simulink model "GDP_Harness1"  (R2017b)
settings: Solver=FixedStepDiscrete  StartTime=0.0  StopTime=2  FixedStep=0.01  RelTol=1e-3  EnableMultiTasking=on
undefined symbols (not defined in the file): sigbuilder_block

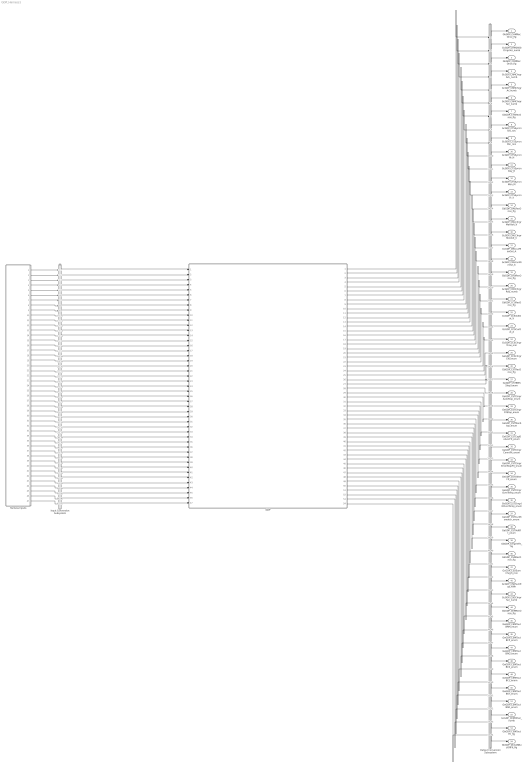
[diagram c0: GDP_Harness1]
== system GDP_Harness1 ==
  GDP : ModelReference  ModelNameDialog=GDP  SimulationMode=Normal  ModelReferenceVersion='M100C100'
  Harness Inputs : Subsystem  Tag=STV Subsys  LoadFcn=sigbuilder_block('load');  StartFcn=sigbuilder_block('start');  StopFcn=sigbuilder_block('stop');  ClipboardFcn=sigbuilder_block('clipboard');  mask(Sigbuilder block){tuvar=[0:10]}
      mask init:
      | if ~strcmp(get_param(bdroot(gcb),'SimulationStatus'),'stopped'),tuvar = sigbuilder_block('maskInit'); end
  Input Conversion Subsystem : Subsystem  Tag=__SLT_ICS__  Description=Signal spec. and routing
  Output Conversion Subsystem : Subsystem  Tag=__SLT_OCS__  Description=Signal spec. and routing
  GbGDP_CHMRecOnce_flg : Outport  OutDataTypeStr=boolean  PortDimensions=[1]
  GcGDP_CHM2600ChrgrVer_numb : Outport  Port=2  OutDataTypeStr=uint32  PortDimensions=[1]
  GbGDP_CRMRecOnce_flg : Outport  Port=3  OutDataTypeStr=boolean  PortDimensions=[1]
  GcGDP_CRMChrgrAck_numb : Outport  Port=4  OutDataTypeStr=uint8  PortDimensions=[1]
  GcGDP_CRMChrgrAr_numb : Outport  Port=5  OutDataTypeStr=uint32  PortDimensions=[1]
  GcGDP_CRMChrgrSer_numb : Outport  Port=6  OutDataTypeStr=uint32  PortDimensions=[1]
  GbGDP_CTSRecOnce_flg : Outport  Port=7  OutDataTypeStr=boolean  PortDimensions=[1]
  GcGDP_CTSSyncnSec_sec : Outport  Port=8  OutDataTypeStr=uint8  PortDimensions=[1]
  GcGDP_CTSSyncnMin_min : Outport  Port=9  OutDataTypeStr=uint8  PortDimensions=[1]
  GcGDP_CTSSyncnHr_H : Outport  Port=10  OutDataTypeStr=uint8  PortDimensions=[1]
  GcGDP_CTSSyncnDay_D : Outport  Port=11  OutDataTypeStr=uint8  PortDimensions=[1]
  GcGDP_CTSSyncnMon_M : Outport  Port=12  OutDataTypeStr=uint8  PortDimensions=[1]
  GcGDP_CTSSyncnYr_Y : Outport  Port=13  OutDataTypeStr=uint16  PortDimensions=[1]
  GbGDP_CMLRecOnce_flg : Outport  Port=14  OutDataTypeStr=boolean  PortDimensions=[1]
  GcGDP_CMLChrgrMaxVolt_V : Outport  Port=15  OutDataTypeStr=single  PortDimensions=[1]
  GcGDP_CMLChrgrMinVolt_V : Outport  Port=16  OutDataTypeStr=single  PortDimensions=[1]
  GcGDP_CMLCurMaxOut_A : Outport  Port=17  OutDataTypeStr=single  PortDimensions=[1]
  GcGDP_CMLCurMinOut_A : Outport  Port=18  OutDataTypeStr=single  PortDimensions=[1]
  GbGDP_CRORecOnce_flg : Outport  Port=19  OutDataTypeStr=boolean  PortDimensions=[1]
  GcGDP_CROChrgrRdy_numb : Outport  Port=20  OutDataTypeStr=uint8  PortDimensions=[1]
  GbGDP_CCSRecOnce_flg : Outport  Port=21  OutDataTypeStr=boolean  PortDimensions=[1]
  GcGDP_CCSVoltOut_V : Outport  Port=22  OutDataTypeStr=single  PortDimensions=[1]
  GcGDP_CCSCurOut_A : Outport  Port=23  OutDataTypeStr=single  PortDimensions=[1]
  GcGDP_CCSChrgrTime_min : Outport  Port=24  OutDataTypeStr=single  PortDimensions=[1]
  GeGDP_CCSChrgrEN_enum : Outport  Port=25  OutDataTypeStr=uint8  PortDimensions=[1]
  GbGDP_CSTRecOnce_flg : Outport  Port=26  OutDataTypeStr=boolean  PortDimensions=[1]
  GeGDP_CSTBMSStop_enum : Outport  Port=27  OutDataTypeStr=uint8  PortDimensions=[1]
  GeGDP_CSTChrgrAutoStop_enum : Outport  Port=28  OutDataTypeStr=uint8  PortDimensions=[1]
  GeGDP_CSTChrgrFltStop_enum : Outport  Port=29  OutDataTypeStr=uint8  PortDimensions=[1]
  GeGDP_CSTManStop_enum : Outport  Port=30  OutDataTypeStr=uint8  PortDimensions=[1]
  GeGDP_CSTCapDeliverFlt_enum : Outport  Port=31  OutDataTypeStr=uint8  PortDimensions=[1]
  GeGDP_CSTChrgrConntFlt_enum : Outport  Port=32  OutDataTypeStr=uint8  PortDimensions=[1]
  GeGDP_CSTChrgrEmerStopFlt_enum : Outport  Port=33  OutDataTypeStr=uint8  PortDimensions=[1]
  GeGDP_CSTOtherFlt_enum : Outport  Port=34  OutDataTypeStr=uint8  PortDimensions=[1]
  GeGDP_CSTChrgrOverTemp_enum : Outport  Port=35  OutDataTypeStr=uint8  PortDimensions=[1]
  GeGDP_CSTChrgrIntOverTemp_enum : Outport  Port=36  OutDataTypeStr=uint8  PortDimensions=[1]
  GeGDP_CSTCurMismatch_enum : Outport  Port=37  OutDataTypeStr=uint8  PortDimensions=[1]
  GeGDP_CSTVoltFlt_enum : Outport  Port=38  OutDataTypeStr=uint8  PortDimensions=[1]
  GbGDP_ChrgrInFlt_flg : Outport  Port=39  OutDataTypeStr=boolean  PortDimensions=[1]
  GbGDP_CSDRecOnce_flg : Outport  Port=40  OutDataTypeStr=boolean  PortDimensions=[1]
  GcGDP_CSDSumChrgTi_min : Outport  Port=41  OutDataTypeStr=single  PortDimensions=[1]
  GcGDP_CSDSumEgy_kWh : Outport  Port=42  OutDataTypeStr=single  PortDimensions=[1]
  GcGDP_CSDChrgrSer_numb : Outport  Port=43  OutDataTypeStr=uint32  PortDimensions=[1]
  GbGDP_CEMRecOnce_flg : Outport  Port=44  OutDataTypeStr=boolean  PortDimensions=[1]
  GeGDP_CEMToutBRM_enum : Outport  Port=45  OutDataTypeStr=uint8  PortDimensions=[1]
  GeGDP_CEMToutBCP_enum : Outport  Port=46  OutDataTypeStr=uint8  PortDimensions=[1]
  GeGDP_CEMToutBRO_enum : Outport  Port=47  OutDataTypeStr=uint8  PortDimensions=[1]
  GeGDP_CEMToutBCS_enum : Outport  Port=48  OutDataTypeStr=uint8  PortDimensions=[1]
  GeGDP_CEMToutBCL_enum : Outport  Port=49  OutDataTypeStr=uint8  PortDimensions=[1]
  GeGDP_CEMToutBST_enum : Outport  Port=50  OutDataTypeStr=uint8  PortDimensions=[1]
  GeGDP_CEMToutBSD_enum : Outport  Port=51  OutDataTypeStr=uint8  PortDimensions=[1]
  GcGDP_CEMOther_numb : Outport  Port=52  OutDataTypeStr=uint8  PortDimensions=[1]
  GbGDP_CEMToutFlt_flg : Outport  Port=53  OutDataTypeStr=boolean  PortDimensions=[1]
  GbGDP_DCCANBusOffFlt_flg : Outport  Port=54  OutDataTypeStr=boolean  PortDimensions=[1]
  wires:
  Harness Inputs/1(GcISP_2600ChrgrVer_numb) -> Input Conversion Subsystem/1(Inport_1)
  Harness Inputs/2(GcISP_2560ChrgrAck_numb) -> Input Conversion Subsystem/2(Inport_2)
  Harness Inputs/3(GcISP_2561ChrgrSer_numb) -> Input Conversion Subsystem/3(Inport_3)
  Harness Inputs/4(GcISP_2562ChrgrAr_numb) -> Input Conversion Subsystem/4(Inport_4)
  Harness Inputs/5(GcISP_2823SyncnSec_sec) -> Input Conversion Subsystem/5(Inport_5)
  Harness Inputs/6(GcISP_2823SyncnMin_min) -> Input Conversion Subsystem/6(Inport_6)
  Harness Inputs/7(GcISP_2823SyncnHr_H) -> Input Conversion Subsystem/7(Inport_7)
  Harness Inputs/8(GcISP_2823SyncnDay_D) -> Input Conversion Subsystem/8(Inport_8)
  Harness Inputs/9(GcISP_2823SyncnMon_M) -> Input Conversion Subsystem/9(Inport_9)
  Harness Inputs/10(GcISP_2823SyncnYr_Y) -> Input Conversion Subsystem/10(Inport_10)
  Harness Inputs/11(GcISP_2824ChrgrMaxVolt_V) -> Input Conversion Subsystem/11(Inport_11)
  Harness Inputs/12(GcISP_2825ChrgrMinVolt_V) -> Input Conversion Subsystem/12(Inport_12)
  Harness Inputs/13(GcISP_2826ChrgrMaxCur_A) -> Input Conversion Subsystem/13(Inport_13)
  Harness Inputs/14(GcISP_2827ChrgrMinCur_A) -> Input Conversion Subsystem/14(Inport_14)
  Harness Inputs/15(GcISP_2830ChrgrRdy_numb) -> Input Conversion Subsystem/15(Inport_15)
  Harness Inputs/16(GcISP_3081ChrgrVolt_V) -> Input Conversion Subsystem/16(Inport_16)
  Harness Inputs/17(GcISP_3082ChrgrCur_A) -> Input Conversion Subsystem/17(Inport_17)
  Harness Inputs/18(GcISP_3083ChrgTi_min) -> Input Conversion Subsystem/18(Inport_18)
  Harness Inputs/19(GeISP_3929ChrgrRdy_enum) -> Input Conversion Subsystem/19(Inport_19)
  Harness Inputs/20(GeISP_3521BMSStop_enum) -> Input Conversion Subsystem/20(Inport_20)
  Harness Inputs/21(GeISP_3521ChrgrAuto_enum) -> Input Conversion Subsystem/21(Inport_21)
  Harness Inputs/22(GeISP_3521ChrgrFlt_enum) -> Input Conversion Subsystem/22(Inport_22)
  Harness Inputs/23(GeISP_3521ManStop_enum) -> Input Conversion Subsystem/23(Inport_23)
  Harness Inputs/24(GeISP_3522CapDeliverFlt_enum) -> Input Conversion Subsystem/24(Inport_24)
  Harness Inputs/25(GeISP_3522ChrgrConntFlt_enum) -> Input Conversion Subsystem/25(Inport_25)
  Harness Inputs/26(GeISP_3522ChrgrEmerStopFlt_enum) -> Input Conversion Subsystem/26(Inport_26)
  Harness Inputs/27(GeISP_3522OtherFlt_enum) -> Input Conversion Subsystem/27(Inport_27)
  Harness Inputs/28(GeISP_3522ChrgrOverTemp_enum) -> Input Conversion Subsystem/28(Inport_28)
  Harness Inputs/29(GeISP_3522ChrgrIntOverTemp_enum) -> Input Conversion Subsystem/29(Inport_29)
  Harness Inputs/30(GeISP_3523CurMismatch_enum) -> Input Conversion Subsystem/30(Inport_30)
  Harness Inputs/31(GeISP_3523VoltFlt_enum) -> Input Conversion Subsystem/31(Inport_31)
  Harness Inputs/32(GcISP_3611SumChrgTi_min) -> Input Conversion Subsystem/32(Inport_32)
  Harness Inputs/33(GcISP_3612SumEgy_kWh) -> Input Conversion Subsystem/33(Inport_33)
  Harness Inputs/34(GcISP_3613ChrgrSer_numb) -> Input Conversion Subsystem/34(Inport_34)
  Harness Inputs/35(GeISP_3921ToutBRM_enum) -> Input Conversion Subsystem/35(Inport_35)
  Harness Inputs/36(GeISP_3922ToutBCP_enum) -> Input Conversion Subsystem/36(Inport_36)
  Harness Inputs/37(GeISP_3923ToutBRO_enum) -> Input Conversion Subsystem/37(Inport_37)
  Harness Inputs/38(GeISP_3924ToutBCS_enum) -> Input Conversion Subsystem/38(Inport_38)
  Harness Inputs/39(GeISP_3925ToutBCL_enum) -> Input Conversion Subsystem/39(Inport_39)
  Harness Inputs/40(GeISP_3926ToutBST_enum) -> Input Conversion Subsystem/40(Inport_40)
  Harness Inputs/41(GeISP_3927ToutBSD_enum) -> Input Conversion Subsystem/41(Inport_41)
  Harness Inputs/42(GcISP_CEMOther_numb) -> Input Conversion Subsystem/42(Inport_42)
  Harness Inputs/43(GeDCC_DCConnSt_enum) -> Input Conversion Subsystem/43(Inport_43)
  Harness Inputs/44(GbISP_DCCANBusOffFlt_flg) -> Input Conversion Subsystem/44(Inport_44)
  Harness Inputs/45(GbISP_DCChrgCanNetStatus_flg) -> Input Conversion Subsystem/45(Inport_45)
  Harness Inputs/46(GeLDP_CC2St_enum) -> Input Conversion Subsystem/46(Inport_46)
  Harness Inputs/47(GbLDP_DC12VSply_flg) -> Input Conversion Subsystem/47(Inport_47)
  Output Conversion Subsystem/1(Outport_1) -> GbGDP_CHMRecOnce_flg/1
  Output Conversion Subsystem/2(Outport_2) -> GcGDP_CHM2600ChrgrVer_numb/1
  Output Conversion Subsystem/3(Outport_3) -> GbGDP_CRMRecOnce_flg/1
  Output Conversion Subsystem/4(Outport_4) -> GcGDP_CRMChrgrAck_numb/1
  Output Conversion Subsystem/5(Outport_5) -> GcGDP_CRMChrgrAr_numb/1
  Output Conversion Subsystem/6(Outport_6) -> GcGDP_CRMChrgrSer_numb/1
  Output Conversion Subsystem/7(Outport_7) -> GbGDP_CTSRecOnce_flg/1
  Output Conversion Subsystem/8(Outport_8) -> GcGDP_CTSSyncnSec_sec/1
  Output Conversion Subsystem/9(Outport_9) -> GcGDP_CTSSyncnMin_min/1
  Output Conversion Subsystem/10(Outport_10) -> GcGDP_CTSSyncnHr_H/1
  Output Conversion Subsystem/11(Outport_11) -> GcGDP_CTSSyncnDay_D/1
  Output Conversion Subsystem/12(Outport_12) -> GcGDP_CTSSyncnMon_M/1
  Output Conversion Subsystem/13(Outport_13) -> GcGDP_CTSSyncnYr_Y/1
  Output Conversion Subsystem/14(Outport_14) -> GbGDP_CMLRecOnce_flg/1
  Output Conversion Subsystem/15(Outport_15) -> GcGDP_CMLChrgrMaxVolt_V/1
  Output Conversion Subsystem/16(Outport_16) -> GcGDP_CMLChrgrMinVolt_V/1
  Output Conversion Subsystem/17(Outport_17) -> GcGDP_CMLCurMaxOut_A/1
  Output Conversion Subsystem/18(Outport_18) -> GcGDP_CMLCurMinOut_A/1
  Output Conversion Subsystem/19(Outport_19) -> GbGDP_CRORecOnce_flg/1
  Output Conversion Subsystem/20(Outport_20) -> GcGDP_CROChrgrRdy_numb/1
  Output Conversion Subsystem/21(Outport_21) -> GbGDP_CCSRecOnce_flg/1
  Output Conversion Subsystem/22(Outport_22) -> GcGDP_CCSVoltOut_V/1
  Output Conversion Subsystem/23(Outport_23) -> GcGDP_CCSCurOut_A/1
  Output Conversion Subsystem/24(Outport_24) -> GcGDP_CCSChrgrTime_min/1
  Output Conversion Subsystem/25(Outport_25) -> GeGDP_CCSChrgrEN_enum/1
  Output Conversion Subsystem/26(Outport_26) -> GbGDP_CSTRecOnce_flg/1
  Output Conversion Subsystem/27(Outport_27) -> GeGDP_CSTBMSStop_enum/1
  Output Conversion Subsystem/28(Outport_28) -> GeGDP_CSTChrgrAutoStop_enum/1
  Output Conversion Subsystem/29(Outport_29) -> GeGDP_CSTChrgrFltStop_enum/1
  Output Conversion Subsystem/30(Outport_30) -> GeGDP_CSTManStop_enum/1
  Output Conversion Subsystem/31(Outport_31) -> GeGDP_CSTCapDeliverFlt_enum/1
  Output Conversion Subsystem/32(Outport_32) -> GeGDP_CSTChrgrConntFlt_enum/1
  Output Conversion Subsystem/33(Outport_33) -> GeGDP_CSTChrgrEmerStopFlt_enum/1
  Output Conversion Subsystem/34(Outport_34) -> GeGDP_CSTOtherFlt_enum/1
  Output Conversion Subsystem/35(Outport_35) -> GeGDP_CSTChrgrOverTemp_enum/1
  Output Conversion Subsystem/36(Outport_36) -> GeGDP_CSTChrgrIntOverTemp_enum/1
  Output Conversion Subsystem/37(Outport_37) -> GeGDP_CSTCurMismatch_enum/1
  Output Conversion Subsystem/38(Outport_38) -> GeGDP_CSTVoltFlt_enum/1
  Output Conversion Subsystem/39(Outport_39) -> GbGDP_ChrgrInFlt_flg/1
  Output Conversion Subsystem/40(Outport_40) -> GbGDP_CSDRecOnce_flg/1
  Output Conversion Subsystem/41(Outport_41) -> GcGDP_CSDSumChrgTi_min/1
  Output Conversion Subsystem/42(Outport_42) -> GcGDP_CSDSumEgy_kWh/1
  Output Conversion Subsystem/43(Outport_43) -> GcGDP_CSDChrgrSer_numb/1
  Output Conversion Subsystem/44(Outport_44) -> GbGDP_CEMRecOnce_flg/1
  Output Conversion Subsystem/45(Outport_45) -> GeGDP_CEMToutBRM_enum/1
  Output Conversion Subsystem/46(Outport_46) -> GeGDP_CEMToutBCP_enum/1
  Output Conversion Subsystem/47(Outport_47) -> GeGDP_CEMToutBRO_enum/1
  Output Conversion Subsystem/48(Outport_48) -> GeGDP_CEMToutBCS_enum/1
  Output Conversion Subsystem/49(Outport_49) -> GeGDP_CEMToutBCL_enum/1
  Output Conversion Subsystem/50(Outport_50) -> GeGDP_CEMToutBST_enum/1
  Output Conversion Subsystem/51(Outport_51) -> GeGDP_CEMToutBSD_enum/1
  Output Conversion Subsystem/52(Outport_52) -> GcGDP_CEMOther_numb/1
  Output Conversion Subsystem/53(Outport_53) -> GbGDP_CEMToutFlt_flg/1
  Output Conversion Subsystem/54(Outport_54) -> GbGDP_DCCANBusOffFlt_flg/1
  Input Conversion Subsystem/1(Outport_1) -> GDP/1
  Input Conversion Subsystem/2(Outport_2) -> GDP/2
  Input Conversion Subsystem/3(Outport_3) -> GDP/3
  Input Conversion Subsystem/4(Outport_4) -> GDP/4
  Input Conversion Subsystem/5(Outport_5) -> GDP/5
  Input Conversion Subsystem/6(Outport_6) -> GDP/6
  Input Conversion Subsystem/7(Outport_7) -> GDP/7
  Input Conversion Subsystem/8(Outport_8) -> GDP/8
  Input Conversion Subsystem/9(Outport_9) -> GDP/9
  Input Conversion Subsystem/10(Outport_10) -> GDP/10
  Input Conversion Subsystem/11(Outport_11) -> GDP/11
  Input Conversion Subsystem/12(Outport_12) -> GDP/12
  Input Conversion Subsystem/13(Outport_13) -> GDP/13
  Input Conversion Subsystem/14(Outport_14) -> GDP/14
  Input Conversion Subsystem/15(Outport_15) -> GDP/15
  Input Conversion Subsystem/16(Outport_16) -> GDP/16
  Input Conversion Subsystem/17(Outport_17) -> GDP/17
  Input Conversion Subsystem/18(Outport_18) -> GDP/18
  Input Conversion Subsystem/19(Outport_19) -> GDP/19
  Input Conversion Subsystem/20(Outport_20) -> GDP/20
  Input Conversion Subsystem/21(Outport_21) -> GDP/21
  Input Conversion Subsystem/22(Outport_22) -> GDP/22
  Input Conversion Subsystem/23(Outport_23) -> GDP/23
  Input Conversion Subsystem/24(Outport_24) -> GDP/24
  Input Conversion Subsystem/25(Outport_25) -> GDP/25
  Input Conversion Subsystem/26(Outport_26) -> GDP/26
  Input Conversion Subsystem/27(Outport_27) -> GDP/27
  Input Conversion Subsystem/28(Outport_28) -> GDP/28
  Input Conversion Subsystem/29(Outport_29) -> GDP/29
  Input Conversion Subsystem/30(Outport_30) -> GDP/30
  Input Conversion Subsystem/31(Outport_31) -> GDP/31
  Input Conversion Subsystem/32(Outport_32) -> GDP/32
  Input Conversion Subsystem/33(Outport_33) -> GDP/33
  Input Conversion Subsystem/34(Outport_34) -> GDP/34
  Input Conversion Subsystem/35(Outport_35) -> GDP/35
  Input Conversion Subsystem/36(Outport_36) -> GDP/36
  Input Conversion Subsystem/37(Outport_37) -> GDP/37
  Input Conversion Subsystem/38(Outport_38) -> GDP/38
  Input Conversion Subsystem/39(Outport_39) -> GDP/39
  Input Conversion Subsystem/40(Outport_40) -> GDP/40
  Input Conversion Subsystem/41(Outport_41) -> GDP/41
  Input Conversion Subsystem/42(Outport_42) -> GDP/42
  Input Conversion Subsystem/43(Outport_43) -> GDP/43
  Input Conversion Subsystem/44(Outport_44) -> GDP/44
  Input Conversion Subsystem/45(Outport_45) -> GDP/45
  Input Conversion Subsystem/46(Outport_46) -> GDP/46
  Input Conversion Subsystem/47(Outport_47) -> GDP/47
  GDP/1 -> Output Conversion Subsystem/1(Inport_1)
  GDP/2 -> Output Conversion Subsystem/2(Inport_2)
  GDP/3 -> Output Conversion Subsystem/3(Inport_3)
  GDP/4 -> Output Conversion Subsystem/4(Inport_4)
  GDP/5 -> Output Conversion Subsystem/5(Inport_5)
  GDP/6 -> Output Conversion Subsystem/6(Inport_6)
  GDP/7 -> Output Conversion Subsystem/7(Inport_7)
  GDP/8 -> Output Conversion Subsystem/8(Inport_8)
  GDP/9 -> Output Conversion Subsystem/9(Inport_9)
  GDP/10 -> Output Conversion Subsystem/10(Inport_10)
  GDP/11 -> Output Conversion Subsystem/11(Inport_11)
  GDP/12 -> Output Conversion Subsystem/12(Inport_12)
  GDP/13 -> Output Conversion Subsystem/13(Inport_13)
  GDP/14 -> Output Conversion Subsystem/14(Inport_14)
  GDP/15 -> Output Conversion Subsystem/15(Inport_15)
  GDP/16 -> Output Conversion Subsystem/16(Inport_16)
  GDP/17 -> Output Conversion Subsystem/17(Inport_17)
  GDP/18 -> Output Conversion Subsystem/18(Inport_18)
  GDP/19 -> Output Conversion Subsystem/19(Inport_19)
  GDP/20 -> Output Conversion Subsystem/20(Inport_20)
  GDP/21 -> Output Conversion Subsystem/21(Inport_21)
  GDP/22 -> Output Conversion Subsystem/22(Inport_22)
  GDP/23 -> Output Conversion Subsystem/23(Inport_23)
  GDP/24 -> Output Conversion Subsystem/24(Inport_24)
  GDP/25 -> Output Conversion Subsystem/25(Inport_25)
  GDP/26 -> Output Conversion Subsystem/26(Inport_26)
  GDP/27 -> Output Conversion Subsystem/27(Inport_27)
  GDP/28 -> Output Conversion Subsystem/28(Inport_28)
  GDP/29 -> Output Conversion Subsystem/29(Inport_29)
  GDP/30 -> Output Conversion Subsystem/30(Inport_30)
  GDP/31 -> Output Conversion Subsystem/31(Inport_31)
  GDP/32 -> Output Conversion Subsystem/32(Inport_32)
  GDP/33 -> Output Conversion Subsystem/33(Inport_33)
  GDP/34 -> Output Conversion Subsystem/34(Inport_34)
  GDP/35 -> Output Conversion Subsystem/35(Inport_35)
  GDP/36 -> Output Conversion Subsystem/36(Inport_36)
  GDP/37 -> Output Conversion Subsystem/37(Inport_37)
  GDP/38 -> Output Conversion Subsystem/38(Inport_38)
  GDP/39 -> Output Conversion Subsystem/39(Inport_39)
  GDP/40 -> Output Conversion Subsystem/40(Inport_40)
  GDP/41 -> Output Conversion Subsystem/41(Inport_41)
  GDP/42 -> Output Conversion Subsystem/42(Inport_42)
  GDP/43 -> Output Conversion Subsystem/43(Inport_43)
  GDP/44 -> Output Conversion Subsystem/44(Inport_44)
  GDP/45 -> Output Conversion Subsystem/45(Inport_45)
  GDP/46 -> Output Conversion Subsystem/46(Inport_46)
  GDP/47 -> Output Conversion Subsystem/47(Inport_47)
  GDP/48 -> Output Conversion Subsystem/48(Inport_48)
  GDP/49 -> Output Conversion Subsystem/49(Inport_49)
  GDP/50 -> Output Conversion Subsystem/50(Inport_50)
  GDP/51 -> Output Conversion Subsystem/51(Inport_51)
  GDP/52 -> Output Conversion Subsystem/52(Inport_52)
  GDP/53 -> Output Conversion Subsystem/53(Inport_53)
  GDP/54 -> Output Conversion Subsystem/54(Inport_54)

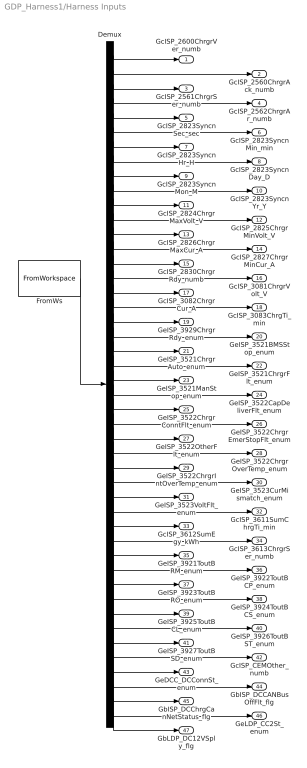
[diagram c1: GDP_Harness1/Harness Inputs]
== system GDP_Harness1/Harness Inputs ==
  Demux : Demux  Tag=STV Demux  Outputs=47
  FromWs : FromWorkspace  Tag=STV FromWs  VariableName=tuvar  SampleTime=0
  GcISP_2600ChrgrVer_numb : Outport  Tag=STV Outport
  GcISP_2560ChrgrAck_numb : Outport  Tag=STV Outport  Port=2
  GcISP_2561ChrgrSer_numb : Outport  Tag=STV Outport  Port=3
  GcISP_2562ChrgrAr_numb : Outport  Tag=STV Outport  Port=4
  GcISP_2823SyncnSec_sec : Outport  Tag=STV Outport  Port=5
  GcISP_2823SyncnMin_min : Outport  Tag=STV Outport  Port=6
  GcISP_2823SyncnHr_H : Outport  Tag=STV Outport  Port=7
  GcISP_2823SyncnDay_D : Outport  Tag=STV Outport  Port=8
  GcISP_2823SyncnMon_M : Outport  Tag=STV Outport  Port=9
  GcISP_2823SyncnYr_Y : Outport  Tag=STV Outport  Port=10
  GcISP_2824ChrgrMaxVolt_V : Outport  Tag=STV Outport  Port=11
  GcISP_2825ChrgrMinVolt_V : Outport  Tag=STV Outport  Port=12
  GcISP_2826ChrgrMaxCur_A : Outport  Tag=STV Outport  Port=13
  GcISP_2827ChrgrMinCur_A : Outport  Tag=STV Outport  Port=14
  GcISP_2830ChrgrRdy_numb : Outport  Tag=STV Outport  Port=15
  GcISP_3081ChrgrVolt_V : Outport  Tag=STV Outport  Port=16
  GcISP_3082ChrgrCur_A : Outport  Tag=STV Outport  Port=17
  GcISP_3083ChrgTi_min : Outport  Tag=STV Outport  Port=18
  GeISP_3929ChrgrRdy_enum : Outport  Tag=STV Outport  Port=19
  GeISP_3521BMSStop_enum : Outport  Tag=STV Outport  Port=20
  GeISP_3521ChrgrAuto_enum : Outport  Tag=STV Outport  Port=21
  GeISP_3521ChrgrFlt_enum : Outport  Tag=STV Outport  Port=22
  GeISP_3521ManStop_enum : Outport  Tag=STV Outport  Port=23
  GeISP_3522CapDeliverFlt_enum : Outport  Tag=STV Outport  Port=24
  GeISP_3522ChrgrConntFlt_enum : Outport  Tag=STV Outport  Port=25
  GeISP_3522ChrgrEmerStopFlt_enum : Outport  Tag=STV Outport  Port=26
  GeISP_3522OtherFlt_enum : Outport  Tag=STV Outport  Port=27
  GeISP_3522ChrgrOverTemp_enum : Outport  Tag=STV Outport  Port=28
  GeISP_3522ChrgrIntOverTemp_enum : Outport  Tag=STV Outport  Port=29
  GeISP_3523CurMismatch_enum : Outport  Tag=STV Outport  Port=30
  GeISP_3523VoltFlt_enum : Outport  Tag=STV Outport  Port=31
  GcISP_3611SumChrgTi_min : Outport  Tag=STV Outport  Port=32
  GcISP_3612SumEgy_kWh : Outport  Tag=STV Outport  Port=33
  GcISP_3613ChrgrSer_numb : Outport  Tag=STV Outport  Port=34
  GeISP_3921ToutBRM_enum : Outport  Tag=STV Outport  Port=35
  GeISP_3922ToutBCP_enum : Outport  Tag=STV Outport  Port=36
  GeISP_3923ToutBRO_enum : Outport  Tag=STV Outport  Port=37
  GeISP_3924ToutBCS_enum : Outport  Tag=STV Outport  Port=38
  GeISP_3925ToutBCL_enum : Outport  Tag=STV Outport  Port=39
  GeISP_3926ToutBST_enum : Outport  Tag=STV Outport  Port=40
  GeISP_3927ToutBSD_enum : Outport  Tag=STV Outport  Port=41
  GcISP_CEMOther_numb : Outport  Tag=STV Outport  Port=42
  GeDCC_DCConnSt_enum : Outport  Tag=STV Outport  Port=43
  GbISP_DCCANBusOffFlt_flg : Outport  Tag=STV Outport  Port=44
  GbISP_DCChrgCanNetStatus_flg : Outport  Tag=STV Outport  Port=45
  GeLDP_CC2St_enum : Outport  Tag=STV Outport  Port=46
  GbLDP_DC12VSply_flg : Outport  Tag=STV Outport  Port=47
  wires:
  FromWs/1 -> Demux/1
  Demux/1 -> GcISP_2600ChrgrVer_numb/1
  Demux/2 -> GcISP_2560ChrgrAck_numb/1
  Demux/3 -> GcISP_2561ChrgrSer_numb/1
  Demux/4 -> GcISP_2562ChrgrAr_numb/1
  Demux/5 -> GcISP_2823SyncnSec_sec/1
  Demux/6 -> GcISP_2823SyncnMin_min/1
  Demux/7 -> GcISP_2823SyncnHr_H/1
  Demux/8 -> GcISP_2823SyncnDay_D/1
  Demux/9 -> GcISP_2823SyncnMon_M/1
  Demux/10 -> GcISP_2823SyncnYr_Y/1
  Demux/11 -> GcISP_2824ChrgrMaxVolt_V/1
  Demux/12 -> GcISP_2825ChrgrMinVolt_V/1
  Demux/13 -> GcISP_2826ChrgrMaxCur_A/1
  Demux/14 -> GcISP_2827ChrgrMinCur_A/1
  Demux/15 -> GcISP_2830ChrgrRdy_numb/1
  Demux/16 -> GcISP_3081ChrgrVolt_V/1
  Demux/17 -> GcISP_3082ChrgrCur_A/1
  Demux/18 -> GcISP_3083ChrgTi_min/1
  Demux/19 -> GeISP_3929ChrgrRdy_enum/1
  Demux/20 -> GeISP_3521BMSStop_enum/1
  Demux/21 -> GeISP_3521ChrgrAuto_enum/1
  Demux/22 -> GeISP_3521ChrgrFlt_enum/1
  Demux/23 -> GeISP_3521ManStop_enum/1
  Demux/24 -> GeISP_3522CapDeliverFlt_enum/1
  Demux/25 -> GeISP_3522ChrgrConntFlt_enum/1
  Demux/26 -> GeISP_3522ChrgrEmerStopFlt_enum/1
  Demux/27 -> GeISP_3522OtherFlt_enum/1
  Demux/28 -> GeISP_3522ChrgrOverTemp_enum/1
  Demux/29 -> GeISP_3522ChrgrIntOverTemp_enum/1
  Demux/30 -> GeISP_3523CurMismatch_enum/1
  Demux/31 -> GeISP_3523VoltFlt_enum/1
  Demux/32 -> GcISP_3611SumChrgTi_min/1
  Demux/33 -> GcISP_3612SumEgy_kWh/1
  Demux/34 -> GcISP_3613ChrgrSer_numb/1
  Demux/35 -> GeISP_3921ToutBRM_enum/1
  Demux/36 -> GeISP_3922ToutBCP_enum/1
  Demux/37 -> GeISP_3923ToutBRO_enum/1
  Demux/38 -> GeISP_3924ToutBCS_enum/1
  Demux/39 -> GeISP_3925ToutBCL_enum/1
  Demux/40 -> GeISP_3926ToutBST_enum/1
  Demux/41 -> GeISP_3927ToutBSD_enum/1
  Demux/42 -> GcISP_CEMOther_numb/1
  Demux/43 -> GeDCC_DCConnSt_enum/1
  Demux/44 -> GbISP_DCCANBusOffFlt_flg/1
  Demux/45 -> GbISP_DCChrgCanNetStatus_flg/1
  Demux/46 -> GeLDP_CC2St_enum/1
  Demux/47 -> GbLDP_DC12VSply_flg/1

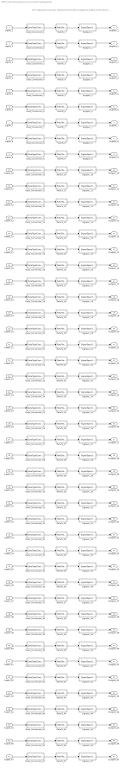
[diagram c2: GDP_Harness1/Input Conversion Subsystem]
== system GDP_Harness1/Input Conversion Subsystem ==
  note: This subsystem has been inserted by Simulink to adapt the output of the source blocks to the interface required by the harnessed component. Modifying the contents of this subsystem may result in compilation and simulation failure.
  Inport_1 : Inport
  Inport_2 : Inport  Port=2
  Inport_3 : Inport  Port=3
  Inport_4 : Inport  Port=4
  Inport_5 : Inport  Port=5
  Inport_6 : Inport  Port=6
  Inport_7 : Inport  Port=7
  Inport_8 : Inport  Port=8
  Inport_9 : Inport  Port=9
  Inport_10 : Inport  Port=10
  Inport_11 : Inport  Port=11
  Inport_12 : Inport  Port=12
  Inport_13 : Inport  Port=13
  Inport_14 : Inport  Port=14
  Inport_15 : Inport  Port=15
  Inport_16 : Inport  Port=16
  Inport_17 : Inport  Port=17
  Inport_18 : Inport  Port=18
  Inport_19 : Inport  Port=19
  Inport_20 : Inport  Port=20
  Inport_21 : Inport  Port=21
  Inport_22 : Inport  Port=22
  Inport_23 : Inport  Port=23
  Inport_24 : Inport  Port=24
  Inport_25 : Inport  Port=25
  Inport_26 : Inport  Port=26
  Inport_27 : Inport  Port=27
  Inport_28 : Inport  Port=28
  Inport_29 : Inport  Port=29
  Inport_30 : Inport  Port=30
  Inport_31 : Inport  Port=31
  Inport_32 : Inport  Port=32
  Inport_33 : Inport  Port=33
  Inport_34 : Inport  Port=34
  Inport_35 : Inport  Port=35
  Inport_36 : Inport  Port=36
  Inport_37 : Inport  Port=37
  Inport_38 : Inport  Port=38
  Inport_39 : Inport  Port=39
  Inport_40 : Inport  Port=40
  Inport_41 : Inport  Port=41
  Inport_42 : Inport  Port=42
  Inport_43 : Inport  Port=43
  Inport_44 : Inport  Port=44
  Inport_45 : Inport  Port=45
  Inport_46 : Inport  Port=46
  Inport_47 : Inport  Port=47
  Data_Conversion_{1,3..4,34} (4 alike) : DataTypeConversion  OutDataTypeStr=uint32
  Data_Conversion_10 : DataTypeConversion  OutDataTypeStr=uint16
  Data_Conversion_{11..12,16,33} (4 alike) : DataTypeConversion  OutDataTypeStr=fixdt('ufix16_Sp1')
  Data_Conversion_13 : DataTypeConversion  OutDataTypeStr=fixdt('ufix16_Sp1_Bn400')
  Data_Conversion_14 : DataTypeConversion  OutDataTypeStr=fixdt('ufix16_Sp1_Bn400')
  Data_Conversion_{2,5..9,15,19..31,35..43,46} (30 alike) : DataTypeConversion  OutDataTypeStr=uint8
  Data_Conversion_17 : DataTypeConversion  OutDataTypeStr=fixdt('ufix16_Sp1_Bn400')
  Data_Conversion_18 : DataTypeConversion  OutDataTypeStr=uint16
  Data_Conversion_32 : DataTypeConversion  OutDataTypeStr=uint16
  Data_Conversion_44 : DataTypeConversion  OutDataTypeStr=boolean
  Data_Conversion_45 : DataTypeConversion  OutDataTypeStr=boolean
  Data_Conversion_47 : DataTypeConversion  OutDataTypeStr=boolean
  RateTs_{1..47} (47 alike) : RateTransition  OutPortSampleTime=0.01
  SigSpec_{1,3..4,34} (4 alike) : SignalSpecification  OutDataTypeStr=uint32  Unit=numb  Dimensions=[1]  SampleTime=0.01
  SigSpec_10 : SignalSpecification  OutDataTypeStr=uint16  Unit=Y  Dimensions=[1]  SampleTime=0.01
  SigSpec_11 : SignalSpecification  OutDataTypeStr=fixdt('ufix16_Sp1')  Unit=V  Dimensions=[1]  SampleTime=0.01
  SigSpec_12 : SignalSpecification  OutDataTypeStr=fixdt('ufix16_Sp1')  Unit=V  Dimensions=[1]  SampleTime=0.01
  SigSpec_13 : SignalSpecification  OutDataTypeStr=fixdt('ufix16_Sp1_Bn400')  Unit=A  Dimensions=[1]  SampleTime=0.01
  SigSpec_14 : SignalSpecification  OutDataTypeStr=fixdt('ufix16_Sp1_Bn400')  Unit=A  Dimensions=[1]  SampleTime=0.01
  SigSpec_15 : SignalSpecification  OutDataTypeStr=uint8  Unit=numb  Dimensions=[1]  SampleTime=0.01
  SigSpec_16 : SignalSpecification  OutDataTypeStr=fixdt('ufix16_Sp1')  Unit=V  Dimensions=[1]  SampleTime=0.01
  SigSpec_17 : SignalSpecification  OutDataTypeStr=fixdt('ufix16_Sp1_Bn400')  Unit=A  Dimensions=[1]  SampleTime=0.01
  SigSpec_18 : SignalSpecification  OutDataTypeStr=uint16  Unit=min  Dimensions=[1]  SampleTime=0.01
  SigSpec_{19..31,35..41,43,46} (22 alike) : SignalSpecification  OutDataTypeStr=uint8  Unit=enum  Dimensions=[1]  SampleTime=0.01
  SigSpec_2 : SignalSpecification  OutDataTypeStr=uint8  Unit=numb  Dimensions=[1]  SampleTime=0.01
  SigSpec_32 : SignalSpecification  OutDataTypeStr=uint16  Unit=min  Dimensions=[1]  SampleTime=0.01
  SigSpec_33 : SignalSpecification  OutDataTypeStr=fixdt('ufix16_Sp1')  Unit=kWh  Dimensions=[1]  SampleTime=0.01
  SigSpec_42 : SignalSpecification  OutDataTypeStr=uint8  Unit=numb  Dimensions=[1]  SampleTime=0.01
  SigSpec_44 : SignalSpecification  OutDataTypeStr=boolean  Unit=flag  Dimensions=[1]  SampleTime=0.01
  SigSpec_45 : SignalSpecification  OutDataTypeStr=boolean  Unit=flag  Dimensions=[1]  SampleTime=0.01
  SigSpec_47 : SignalSpecification  OutDataTypeStr=boolean  Unit=flag  Dimensions=[1]  SampleTime=0.01
  SigSpec_5 : SignalSpecification  OutDataTypeStr=uint8  Unit=sec  Dimensions=[1]  SampleTime=0.01
  SigSpec_6 : SignalSpecification  OutDataTypeStr=uint8  Unit=min  Dimensions=[1]  SampleTime=0.01
  SigSpec_7 : SignalSpecification  OutDataTypeStr=uint8  Unit=H  Dimensions=[1]  SampleTime=0.01
  SigSpec_8 : SignalSpecification  OutDataTypeStr=uint8  Unit=D  Dimensions=[1]  SampleTime=0.01
  SigSpec_9 : SignalSpecification  OutDataTypeStr=uint8  Unit=M  Dimensions=[1]  SampleTime=0.01
  Outport_1 : Outport
  Outport_2 : Outport  Port=2
  Outport_3 : Outport  Port=3
  Outport_4 : Outport  Port=4
  Outport_5 : Outport  Port=5
  Outport_6 : Outport  Port=6
  Outport_7 : Outport  Port=7
  Outport_8 : Outport  Port=8
  Outport_9 : Outport  Port=9
  Outport_10 : Outport  Port=10
  Outport_11 : Outport  Port=11
  Outport_12 : Outport  Port=12
  Outport_13 : Outport  Port=13
  Outport_14 : Outport  Port=14
  Outport_15 : Outport  Port=15
  Outport_16 : Outport  Port=16
  Outport_17 : Outport  Port=17
  Outport_18 : Outport  Port=18
  Outport_19 : Outport  Port=19
  Outport_20 : Outport  Port=20
  Outport_21 : Outport  Port=21
  Outport_22 : Outport  Port=22
  Outport_23 : Outport  Port=23
  Outport_24 : Outport  Port=24
  Outport_25 : Outport  Port=25
  Outport_26 : Outport  Port=26
  Outport_27 : Outport  Port=27
  Outport_28 : Outport  Port=28
  Outport_29 : Outport  Port=29
  Outport_30 : Outport  Port=30
  Outport_31 : Outport  Port=31
  Outport_32 : Outport  Port=32
  Outport_33 : Outport  Port=33
  Outport_34 : Outport  Port=34
  Outport_35 : Outport  Port=35
  Outport_36 : Outport  Port=36
  Outport_37 : Outport  Port=37
  Outport_38 : Outport  Port=38
  Outport_39 : Outport  Port=39
  Outport_40 : Outport  Port=40
  Outport_41 : Outport  Port=41
  Outport_42 : Outport  Port=42
  Outport_43 : Outport  Port=43
  Outport_44 : Outport  Port=44
  Outport_45 : Outport  Port=45
  Outport_46 : Outport  Port=46
  Outport_47 : Outport  Port=47
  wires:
  SigSpec_1/1 -> Outport_1/1
  RateTs_1/1 -> SigSpec_1/1
  Data_Conversion_1/1 -> RateTs_1/1
  Inport_1/1 -> Data_Conversion_1/1
  SigSpec_2/1 -> Outport_2/1
  RateTs_2/1 -> SigSpec_2/1
  Data_Conversion_2/1 -> RateTs_2/1
  Inport_2/1 -> Data_Conversion_2/1
  SigSpec_3/1 -> Outport_3/1
  RateTs_3/1 -> SigSpec_3/1
  Data_Conversion_3/1 -> RateTs_3/1
  Inport_3/1 -> Data_Conversion_3/1
  SigSpec_4/1 -> Outport_4/1
  RateTs_4/1 -> SigSpec_4/1
  Data_Conversion_4/1 -> RateTs_4/1
  Inport_4/1 -> Data_Conversion_4/1
  SigSpec_5/1 -> Outport_5/1
  RateTs_5/1 -> SigSpec_5/1
  Data_Conversion_5/1 -> RateTs_5/1
  Inport_5/1 -> Data_Conversion_5/1
  SigSpec_6/1 -> Outport_6/1
  RateTs_6/1 -> SigSpec_6/1
  Data_Conversion_6/1 -> RateTs_6/1
  Inport_6/1 -> Data_Conversion_6/1
  SigSpec_7/1 -> Outport_7/1
  RateTs_7/1 -> SigSpec_7/1
  Data_Conversion_7/1 -> RateTs_7/1
  Inport_7/1 -> Data_Conversion_7/1
  SigSpec_8/1 -> Outport_8/1
  RateTs_8/1 -> SigSpec_8/1
  Data_Conversion_8/1 -> RateTs_8/1
  Inport_8/1 -> Data_Conversion_8/1
  SigSpec_9/1 -> Outport_9/1
  RateTs_9/1 -> SigSpec_9/1
  Data_Conversion_9/1 -> RateTs_9/1
  Inport_9/1 -> Data_Conversion_9/1
  SigSpec_10/1 -> Outport_10/1
  RateTs_10/1 -> SigSpec_10/1
  Data_Conversion_10/1 -> RateTs_10/1
  Inport_10/1 -> Data_Conversion_10/1
  SigSpec_11/1 -> Outport_11/1
  RateTs_11/1 -> SigSpec_11/1
  Data_Conversion_11/1 -> RateTs_11/1
  Inport_11/1 -> Data_Conversion_11/1
  SigSpec_12/1 -> Outport_12/1
  RateTs_12/1 -> SigSpec_12/1
  Data_Conversion_12/1 -> RateTs_12/1
  Inport_12/1 -> Data_Conversion_12/1
  SigSpec_13/1 -> Outport_13/1
  RateTs_13/1 -> SigSpec_13/1
  Data_Conversion_13/1 -> RateTs_13/1
  Inport_13/1 -> Data_Conversion_13/1
  SigSpec_14/1 -> Outport_14/1
  RateTs_14/1 -> SigSpec_14/1
  Data_Conversion_14/1 -> RateTs_14/1
  Inport_14/1 -> Data_Conversion_14/1
  SigSpec_15/1 -> Outport_15/1
  RateTs_15/1 -> SigSpec_15/1
  Data_Conversion_15/1 -> RateTs_15/1
  Inport_15/1 -> Data_Conversion_15/1
  SigSpec_16/1 -> Outport_16/1
  RateTs_16/1 -> SigSpec_16/1
  Data_Conversion_16/1 -> RateTs_16/1
  Inport_16/1 -> Data_Conversion_16/1
  SigSpec_17/1 -> Outport_17/1
  RateTs_17/1 -> SigSpec_17/1
  Data_Conversion_17/1 -> RateTs_17/1
  Inport_17/1 -> Data_Conversion_17/1
  SigSpec_18/1 -> Outport_18/1
  RateTs_18/1 -> SigSpec_18/1
  Data_Conversion_18/1 -> RateTs_18/1
  Inport_18/1 -> Data_Conversion_18/1
  SigSpec_19/1 -> Outport_19/1
  RateTs_19/1 -> SigSpec_19/1
  Data_Conversion_19/1 -> RateTs_19/1
  Inport_19/1 -> Data_Conversion_19/1
  SigSpec_20/1 -> Outport_20/1
  RateTs_20/1 -> SigSpec_20/1
  Data_Conversion_20/1 -> RateTs_20/1
  Inport_20/1 -> Data_Conversion_20/1
  SigSpec_21/1 -> Outport_21/1
  RateTs_21/1 -> SigSpec_21/1
  Data_Conversion_21/1 -> RateTs_21/1
  Inport_21/1 -> Data_Conversion_21/1
  SigSpec_22/1 -> Outport_22/1
  RateTs_22/1 -> SigSpec_22/1
  Data_Conversion_22/1 -> RateTs_22/1
  Inport_22/1 -> Data_Conversion_22/1
  SigSpec_23/1 -> Outport_23/1
  RateTs_23/1 -> SigSpec_23/1
  Data_Conversion_23/1 -> RateTs_23/1
  Inport_23/1 -> Data_Conversion_23/1
  SigSpec_24/1 -> Outport_24/1
  RateTs_24/1 -> SigSpec_24/1
  Data_Conversion_24/1 -> RateTs_24/1
  Inport_24/1 -> Data_Conversion_24/1
  SigSpec_25/1 -> Outport_25/1
  RateTs_25/1 -> SigSpec_25/1
  Data_Conversion_25/1 -> RateTs_25/1
  Inport_25/1 -> Data_Conversion_25/1
  SigSpec_26/1 -> Outport_26/1
  RateTs_26/1 -> SigSpec_26/1
  Data_Conversion_26/1 -> RateTs_26/1
  Inport_26/1 -> Data_Conversion_26/1
  SigSpec_27/1 -> Outport_27/1
  RateTs_27/1 -> SigSpec_27/1
  Data_Conversion_27/1 -> RateTs_27/1
  Inport_27/1 -> Data_Conversion_27/1
  SigSpec_28/1 -> Outport_28/1
  RateTs_28/1 -> SigSpec_28/1
  Data_Conversion_28/1 -> RateTs_28/1
  Inport_28/1 -> Data_Conversion_28/1
  SigSpec_29/1 -> Outport_29/1
  RateTs_29/1 -> SigSpec_29/1
  Data_Conversion_29/1 -> RateTs_29/1
  Inport_29/1 -> Data_Conversion_29/1
  SigSpec_30/1 -> Outport_30/1
  RateTs_30/1 -> SigSpec_30/1
  Data_Conversion_30/1 -> RateTs_30/1
  Inport_30/1 -> Data_Conversion_30/1
  SigSpec_31/1 -> Outport_31/1
  RateTs_31/1 -> SigSpec_31/1
  Data_Conversion_31/1 -> RateTs_31/1
  Inport_31/1 -> Data_Conversion_31/1
  SigSpec_32/1 -> Outport_32/1
  RateTs_32/1 -> SigSpec_32/1
  Data_Conversion_32/1 -> RateTs_32/1
  Inport_32/1 -> Data_Conversion_32/1
  SigSpec_33/1 -> Outport_33/1
  RateTs_33/1 -> SigSpec_33/1
  Data_Conversion_33/1 -> RateTs_33/1
  Inport_33/1 -> Data_Conversion_33/1
  SigSpec_34/1 -> Outport_34/1
  RateTs_34/1 -> SigSpec_34/1
  Data_Conversion_34/1 -> RateTs_34/1
  Inport_34/1 -> Data_Conversion_34/1
  SigSpec_35/1 -> Outport_35/1
  RateTs_35/1 -> SigSpec_35/1
  Data_Conversion_35/1 -> RateTs_35/1
  Inport_35/1 -> Data_Conversion_35/1
  SigSpec_36/1 -> Outport_36/1
  RateTs_36/1 -> SigSpec_36/1
  Data_Conversion_36/1 -> RateTs_36/1
  Inport_36/1 -> Data_Conversion_36/1
  SigSpec_37/1 -> Outport_37/1
  RateTs_37/1 -> SigSpec_37/1
  Data_Conversion_37/1 -> RateTs_37/1
  Inport_37/1 -> Data_Conversion_37/1
  SigSpec_38/1 -> Outport_38/1
  RateTs_38/1 -> SigSpec_38/1
  Data_Conversion_38/1 -> RateTs_38/1
  Inport_38/1 -> Data_Conversion_38/1
  SigSpec_39/1 -> Outport_39/1
  RateTs_39/1 -> SigSpec_39/1
  Data_Conversion_39/1 -> RateTs_39/1
  Inport_39/1 -> Data_Conversion_39/1
  SigSpec_40/1 -> Outport_40/1
  RateTs_40/1 -> SigSpec_40/1
  Data_Conversion_40/1 -> RateTs_40/1
  Inport_40/1 -> Data_Conversion_40/1
  SigSpec_41/1 -> Outport_41/1
  RateTs_41/1 -> SigSpec_41/1
  Data_Conversion_41/1 -> RateTs_41/1
  Inport_41/1 -> Data_Conversion_41/1
  SigSpec_42/1 -> Outport_42/1
  RateTs_42/1 -> SigSpec_42/1
  Data_Conversion_42/1 -> RateTs_42/1
  Inport_42/1 -> Data_Conversion_42/1
  SigSpec_43/1 -> Outport_43/1
  RateTs_43/1 -> SigSpec_43/1
  Data_Conversion_43/1 -> RateTs_43/1
  Inport_43/1 -> Data_Conversion_43/1
  SigSpec_44/1 -> Outport_44/1
  RateTs_44/1 -> SigSpec_44/1
  Data_Conversion_44/1 -> RateTs_44/1
  Inport_44/1 -> Data_Conversion_44/1
  SigSpec_45/1 -> Outport_45/1
  RateTs_45/1 -> SigSpec_45/1
  Data_Conversion_45/1 -> RateTs_45/1
  Inport_45/1 -> Data_Conversion_45/1
  SigSpec_46/1 -> Outport_46/1
  RateTs_46/1 -> SigSpec_46/1
  Data_Conversion_46/1 -> RateTs_46/1
  Inport_46/1 -> Data_Conversion_46/1
  SigSpec_47/1 -> Outport_47/1
  RateTs_47/1 -> SigSpec_47/1
  Data_Conversion_47/1 -> RateTs_47/1
  Inport_47/1 -> Data_Conversion_47/1

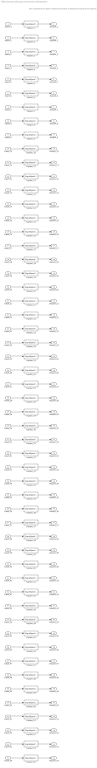
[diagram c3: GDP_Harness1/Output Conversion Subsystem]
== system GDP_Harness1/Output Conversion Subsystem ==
  note: This subsystem has been inserted by Simulink to adapt the output of the harnessed component to the interface required by the sink blocks. Modifying the contents of this subsystem may result in compilation and simulation failure.
  Inport_1 : Inport
  Inport_2 : Inport  Port=2
  Inport_3 : Inport  Port=3
  Inport_4 : Inport  Port=4
  Inport_5 : Inport  Port=5
  Inport_6 : Inport  Port=6
  Inport_7 : Inport  Port=7
  Inport_8 : Inport  Port=8
  Inport_9 : Inport  Port=9
  Inport_10 : Inport  Port=10
  Inport_11 : Inport  Port=11
  Inport_12 : Inport  Port=12
  Inport_13 : Inport  Port=13
  Inport_14 : Inport  Port=14
  Inport_15 : Inport  Port=15
  Inport_16 : Inport  Port=16
  Inport_17 : Inport  Port=17
  Inport_18 : Inport  Port=18
  Inport_19 : Inport  Port=19
  Inport_20 : Inport  Port=20
  Inport_21 : Inport  Port=21
  Inport_22 : Inport  Port=22
  Inport_23 : Inport  Port=23
  Inport_24 : Inport  Port=24
  Inport_25 : Inport  Port=25
  Inport_26 : Inport  Port=26
  Inport_27 : Inport  Port=27
  Inport_28 : Inport  Port=28
  Inport_29 : Inport  Port=29
  Inport_30 : Inport  Port=30
  Inport_31 : Inport  Port=31
  Inport_32 : Inport  Port=32
  Inport_33 : Inport  Port=33
  Inport_34 : Inport  Port=34
  Inport_35 : Inport  Port=35
  Inport_36 : Inport  Port=36
  Inport_37 : Inport  Port=37
  Inport_38 : Inport  Port=38
  Inport_39 : Inport  Port=39
  Inport_40 : Inport  Port=40
  Inport_41 : Inport  Port=41
  Inport_42 : Inport  Port=42
  Inport_43 : Inport  Port=43
  Inport_44 : Inport  Port=44
  Inport_45 : Inport  Port=45
  Inport_46 : Inport  Port=46
  Inport_47 : Inport  Port=47
  Inport_48 : Inport  Port=48
  Inport_49 : Inport  Port=49
  Inport_50 : Inport  Port=50
  Inport_51 : Inport  Port=51
  Inport_52 : Inport  Port=52
  Inport_53 : Inport  Port=53
  Inport_54 : Inport  Port=54
  SigSpec_{1,3,7,14,19,21,26,39..40,44,53..54} (12 alike) : SignalSpecification  OutDataTypeStr=boolean  Unit=flag  Dimensions=[1]  SampleTime=0.01
  SigSpec_10 : SignalSpecification  OutDataTypeStr=uint8  Unit=H  Dimensions=[1]  SampleTime=0.01
  SigSpec_11 : SignalSpecification  OutDataTypeStr=uint8  Unit=D  Dimensions=[1]  SampleTime=0.01
  SigSpec_12 : SignalSpecification  OutDataTypeStr=uint8  Unit=M  Dimensions=[1]  SampleTime=0.01
  SigSpec_13 : SignalSpecification  OutDataTypeStr=uint16  Unit=Y  Dimensions=[1]  SampleTime=0.01
  SigSpec_15 : SignalSpecification  OutDataTypeStr=single  Unit=V  Dimensions=[1]  SampleTime=0.01
  SigSpec_16 : SignalSpecification  OutDataTypeStr=single  Unit=V  Dimensions=[1]  SampleTime=0.01
  SigSpec_17 : SignalSpecification  OutDataTypeStr=single  Unit=A  Dimensions=[1]  SampleTime=0.01
  SigSpec_18 : SignalSpecification  OutDataTypeStr=single  Unit=A  Dimensions=[1]  SampleTime=0.01
  SigSpec_{2,5..6,43} (4 alike) : SignalSpecification  OutDataTypeStr=uint32  Unit=numb  Dimensions=[1]  SampleTime=0.01
  SigSpec_20 : SignalSpecification  OutDataTypeStr=uint8  Unit=numb  Dimensions=[1]  SampleTime=0.01
  SigSpec_22 : SignalSpecification  OutDataTypeStr=single  Unit=V  Dimensions=[1]  SampleTime=0.01
  SigSpec_23 : SignalSpecification  OutDataTypeStr=single  Unit=A  Dimensions=[1]  SampleTime=0.01
  SigSpec_24 : SignalSpecification  OutDataTypeStr=single  Unit=min  Dimensions=[1]  SampleTime=0.01
  SigSpec_{25,27..38,45..51} (20 alike) : SignalSpecification  OutDataTypeStr=uint8  Unit=enum  Dimensions=[1]  SampleTime=0.01
  SigSpec_4 : SignalSpecification  OutDataTypeStr=uint8  Unit=numb  Dimensions=[1]  SampleTime=0.01
  SigSpec_41 : SignalSpecification  OutDataTypeStr=single  Unit=min  Dimensions=[1]  SampleTime=0.01
  SigSpec_42 : SignalSpecification  OutDataTypeStr=single  Unit=kWh  Dimensions=[1]  SampleTime=0.01
  SigSpec_52 : SignalSpecification  OutDataTypeStr=uint8  Unit=numb  Dimensions=[1]  SampleTime=0.01
  SigSpec_8 : SignalSpecification  OutDataTypeStr=uint8  Unit=sec  Dimensions=[1]  SampleTime=0.01
  SigSpec_9 : SignalSpecification  OutDataTypeStr=uint8  Unit=min  Dimensions=[1]  SampleTime=0.01
  Outport_1 : Outport
  Outport_2 : Outport  Port=2
  Outport_3 : Outport  Port=3
  Outport_4 : Outport  Port=4
  Outport_5 : Outport  Port=5
  Outport_6 : Outport  Port=6
  Outport_7 : Outport  Port=7
  Outport_8 : Outport  Port=8
  Outport_9 : Outport  Port=9
  Outport_10 : Outport  Port=10
  Outport_11 : Outport  Port=11
  Outport_12 : Outport  Port=12
  Outport_13 : Outport  Port=13
  Outport_14 : Outport  Port=14
  Outport_15 : Outport  Port=15
  Outport_16 : Outport  Port=16
  Outport_17 : Outport  Port=17
  Outport_18 : Outport  Port=18
  Outport_19 : Outport  Port=19
  Outport_20 : Outport  Port=20
  Outport_21 : Outport  Port=21
  Outport_22 : Outport  Port=22
  Outport_23 : Outport  Port=23
  Outport_24 : Outport  Port=24
  Outport_25 : Outport  Port=25
  Outport_26 : Outport  Port=26
  Outport_27 : Outport  Port=27
  Outport_28 : Outport  Port=28
  Outport_29 : Outport  Port=29
  Outport_30 : Outport  Port=30
  Outport_31 : Outport  Port=31
  Outport_32 : Outport  Port=32
  Outport_33 : Outport  Port=33
  Outport_34 : Outport  Port=34
  Outport_35 : Outport  Port=35
  Outport_36 : Outport  Port=36
  Outport_37 : Outport  Port=37
  Outport_38 : Outport  Port=38
  Outport_39 : Outport  Port=39
  Outport_40 : Outport  Port=40
  Outport_41 : Outport  Port=41
  Outport_42 : Outport  Port=42
  Outport_43 : Outport  Port=43
  Outport_44 : Outport  Port=44
  Outport_45 : Outport  Port=45
  Outport_46 : Outport  Port=46
  Outport_47 : Outport  Port=47
  Outport_48 : Outport  Port=48
  Outport_49 : Outport  Port=49
  Outport_50 : Outport  Port=50
  Outport_51 : Outport  Port=51
  Outport_52 : Outport  Port=52
  Outport_53 : Outport  Port=53
  Outport_54 : Outport  Port=54
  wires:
  Inport_1/1 -> SigSpec_1/1
  SigSpec_1/1 -> Outport_1/1
  Inport_2/1 -> SigSpec_2/1
  SigSpec_2/1 -> Outport_2/1
  Inport_3/1 -> SigSpec_3/1
  SigSpec_3/1 -> Outport_3/1
  Inport_4/1 -> SigSpec_4/1
  SigSpec_4/1 -> Outport_4/1
  Inport_5/1 -> SigSpec_5/1
  SigSpec_5/1 -> Outport_5/1
  Inport_6/1 -> SigSpec_6/1
  SigSpec_6/1 -> Outport_6/1
  Inport_7/1 -> SigSpec_7/1
  SigSpec_7/1 -> Outport_7/1
  Inport_8/1 -> SigSpec_8/1
  SigSpec_8/1 -> Outport_8/1
  Inport_9/1 -> SigSpec_9/1
  SigSpec_9/1 -> Outport_9/1
  Inport_10/1 -> SigSpec_10/1
  SigSpec_10/1 -> Outport_10/1
  Inport_11/1 -> SigSpec_11/1
  SigSpec_11/1 -> Outport_11/1
  Inport_12/1 -> SigSpec_12/1
  SigSpec_12/1 -> Outport_12/1
  Inport_13/1 -> SigSpec_13/1
  SigSpec_13/1 -> Outport_13/1
  Inport_14/1 -> SigSpec_14/1
  SigSpec_14/1 -> Outport_14/1
  Inport_15/1 -> SigSpec_15/1
  SigSpec_15/1 -> Outport_15/1
  Inport_16/1 -> SigSpec_16/1
  SigSpec_16/1 -> Outport_16/1
  Inport_17/1 -> SigSpec_17/1
  SigSpec_17/1 -> Outport_17/1
  Inport_18/1 -> SigSpec_18/1
  SigSpec_18/1 -> Outport_18/1
  Inport_19/1 -> SigSpec_19/1
  SigSpec_19/1 -> Outport_19/1
  Inport_20/1 -> SigSpec_20/1
  SigSpec_20/1 -> Outport_20/1
  Inport_21/1 -> SigSpec_21/1
  SigSpec_21/1 -> Outport_21/1
  Inport_22/1 -> SigSpec_22/1
  SigSpec_22/1 -> Outport_22/1
  Inport_23/1 -> SigSpec_23/1
  SigSpec_23/1 -> Outport_23/1
  Inport_24/1 -> SigSpec_24/1
  SigSpec_24/1 -> Outport_24/1
  Inport_25/1 -> SigSpec_25/1
  SigSpec_25/1 -> Outport_25/1
  Inport_26/1 -> SigSpec_26/1
  SigSpec_26/1 -> Outport_26/1
  Inport_27/1 -> SigSpec_27/1
  SigSpec_27/1 -> Outport_27/1
  Inport_28/1 -> SigSpec_28/1
  SigSpec_28/1 -> Outport_28/1
  Inport_29/1 -> SigSpec_29/1
  SigSpec_29/1 -> Outport_29/1
  Inport_30/1 -> SigSpec_30/1
  SigSpec_30/1 -> Outport_30/1
  Inport_31/1 -> SigSpec_31/1
  SigSpec_31/1 -> Outport_31/1
  Inport_32/1 -> SigSpec_32/1
  SigSpec_32/1 -> Outport_32/1
  Inport_33/1 -> SigSpec_33/1
  SigSpec_33/1 -> Outport_33/1
  Inport_34/1 -> SigSpec_34/1
  SigSpec_34/1 -> Outport_34/1
  Inport_35/1 -> SigSpec_35/1
  SigSpec_35/1 -> Outport_35/1
  Inport_36/1 -> SigSpec_36/1
  SigSpec_36/1 -> Outport_36/1
  Inport_37/1 -> SigSpec_37/1
  SigSpec_37/1 -> Outport_37/1
  Inport_38/1 -> SigSpec_38/1
  SigSpec_38/1 -> Outport_38/1
  Inport_39/1 -> SigSpec_39/1
  SigSpec_39/1 -> Outport_39/1
  Inport_40/1 -> SigSpec_40/1
  SigSpec_40/1 -> Outport_40/1
  Inport_41/1 -> SigSpec_41/1
  SigSpec_41/1 -> Outport_41/1
  Inport_42/1 -> SigSpec_42/1
  SigSpec_42/1 -> Outport_42/1
  Inport_43/1 -> SigSpec_43/1
  SigSpec_43/1 -> Outport_43/1
  Inport_44/1 -> SigSpec_44/1
  SigSpec_44/1 -> Outport_44/1
  Inport_45/1 -> SigSpec_45/1
  SigSpec_45/1 -> Outport_45/1
  Inport_46/1 -> SigSpec_46/1
  SigSpec_46/1 -> Outport_46/1
  Inport_47/1 -> SigSpec_47/1
  SigSpec_47/1 -> Outport_47/1
  Inport_48/1 -> SigSpec_48/1
  SigSpec_48/1 -> Outport_48/1
  Inport_49/1 -> SigSpec_49/1
  SigSpec_49/1 -> Outport_49/1
  Inport_50/1 -> SigSpec_50/1
  SigSpec_50/1 -> Outport_50/1
  Inport_51/1 -> SigSpec_51/1
  SigSpec_51/1 -> Outport_51/1
  Inport_52/1 -> SigSpec_52/1
  SigSpec_52/1 -> Outport_52/1
  Inport_53/1 -> SigSpec_53/1
  SigSpec_53/1 -> Outport_53/1
  Inport_54/1 -> SigSpec_54/1
  SigSpec_54/1 -> Outport_54/1
